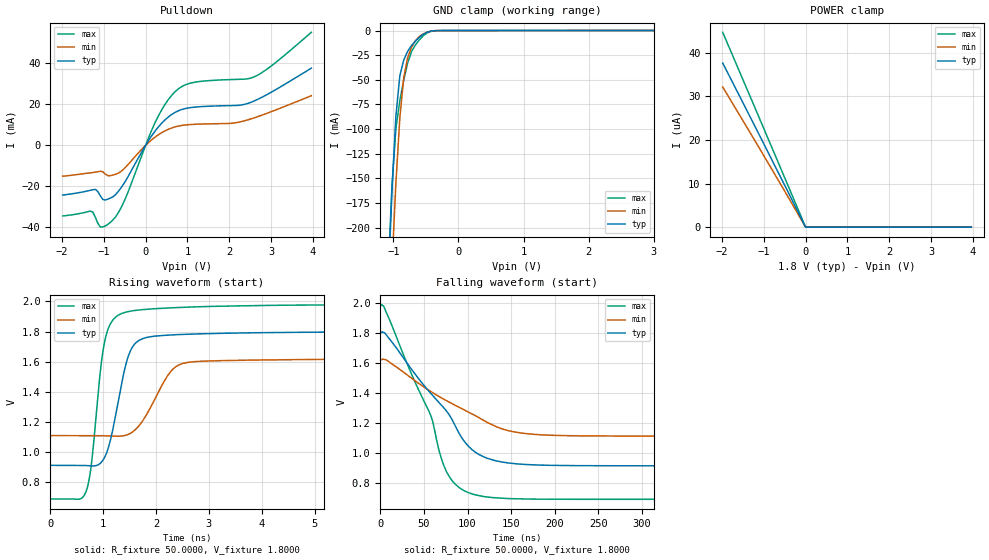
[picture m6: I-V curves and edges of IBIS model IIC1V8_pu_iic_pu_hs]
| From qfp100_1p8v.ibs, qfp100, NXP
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[Model] IIC1V8_pu_iic_pu_hs
|   Model IIC1V8_pu_iic_pu_hs
| This model was characterised for following simulation conditions:
| External (pad) voltage:
|   - Typ: 1.8V,   - Min: 1.62V,   - Max: 1.98V
| Library cells for typ/min/max conditions are connected as defined below:
|  IO - External Pad
|  A - Core Input
|  EN - Output Buffer Enable
|  BOOST - vdde
|  ECS - vdd
|  EGP - gnd
|  ENZI - vdd
|  EPD - gnd
|  EPUN - gnd
|  SSEL - vdd
|  ZI - NC
|  ZIF - NC
|  gnd - gnd
|  gnde - gnde
|  vdd - vdd
|  vdde - vdde
| All other pins connected to ground
Model_type I/O_open_drain
Polarity   Non-Inverting
Enable   Active-Low
Vinl =   0.5400V
Vinh =   1.2600V
Vmeas =  0.9000V
Cref =   0.0F
Rref =   1000.000
Vref =   1.8000V
C_comp   3.6100pF   3.4623pF   3.7513pF
|C_comp_pullup   0.9280pF   0.9063pF   0.9342pF
|C_comp_pulldown   2.3312pF   2.4847pF   2.1853pF
[Model Spec]
| variable   typ   min   max
Vinh   0.5400V   0.4860V   0.5940V
Vinl   1.2600V   1.1340V   1.3860V
Vmeas   0.9000V   0.8100V   0.9900V
Vref   1.8000V   1.6200V   1.9800V
Cref   0.0F   0.0F   0.0F
Rref   1.0000k   1.0000k   1.0000k
[Temperature Range]   25.0000   0.1250k   -40.0000
[Voltage Range]   1.8000V   1.6200V   1.9800V
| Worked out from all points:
|   slope of the pulldown table from 0 to 0.27 V, typ, clamps not added: 33.4 ohm
|   GND clamp passes 1 mA (typ) near -0.44 V on its own axis
|   rising waveform, R_fixture 50.0000, V_fixture 1.8000: 20-80 % time 318ps typ, 486ps min, 235ps max; typ from 0.912 V to 1.8 V
|   falling waveform, R_fixture 50.0000, V_fixture 1.8000: 20-80 % time 67ns typ, 88.7ns min, 48.9ns max; typ from 1.8 V to 0.912 V
[Pulldown]
|Voltage   I(typ)   I(min)   I(max)
-1.98V    -24.22mA   -15.04mA   -34.42mA
-1.32V    -21.94mA   -13.4mA    -32.06mA
-1.2V     -21.45mA   -13.05mA   -35.06mA
-1.08V    -24.63mA   -12.6mA    -39.9mA
-900mV    -26.23mA   -14.78mA   -38.53mA
-720mV    -24.07mA   -14.13mA   -34.99mA
-540mV    -19.33mA   -11.9mA    -28.53mA
300mV     8.856mA    5.096mA    14.12mA
720mV     16.26mA    9.117mA    26.48mA
1.14V     18.6mA     10.26mA    30.69mA
2.58V     21.55mA    13.34mA    33.32mA
3.96V     37.7mA     24.26mA    55.17mA
[GND_clamp]
|Voltage   I(typ)   I(min)   I(max)
-1.98V    -2.104A    -2.075A    -2.136A
-1.08V    -259.3mA   -333mA     -247mA
-1.02V    -161.8mA   -238.7mA   -157.2mA
-960mV    -86.78mA   -154.8mA   -99.51mA
-900mV    -45.99mA   -88.85mA   -71.1mA
-840mV    -29.94mA   -48.03mA   -50.31mA
-780mV    -21.2mA    -27.67mA   -33.04mA
-720mV    -15.2mA    -16.91mA   -21.32mA
-660mV    -10.61mA   -10.27mA   -14.61mA
-540mV    -3.83mA    -3.432mA   -5.346mA
-300mV    -56.31uA   -67.68uA   -68.13uA
3.96V     0A         0A         0A
[POWER_clamp]
|Voltage   I(typ)   I(min)   I(max)
-1.98V    37.59uA    32.11uA    44.63uA
-960mV    18.36uA    15.76uA    21.73uA
0V        104.7pA    4.893nA    11.38pA
3.96V     0A         0A         0A
[Ramp]
| variable   typ   min   max
dV/dt_r  0.5330/0.3182n   0.3064/0.4861n   0.7749/0.2348n
dV/dt_f  0.5329/66.9839n   0.3063/88.7255n   0.7748/48.9516n
R_load = 50.0000
[Rising Waveform]
R_fixture= 50.0000
V_fixture= 1.8000
V_fixture_min= 1.6200
V_fixture_max= 1.9800
|time   V(typ)   V(min)   V(max)
0s        911.7mV    1.109V     688.6mV
674.8ps   910.4mV    1.109V     735.9mV
774.1ps   908mV      1.11V      909mV
1.008ns   952.4mV    1.108V     1.696V
1.271ns   1.309V     1.105V     1.906V
1.478ns   1.64V      1.118V     1.933V
1.767ns   1.756V     1.218V     1.947V
2.535ns   1.782V     1.591V     1.962V
5.946ns   1.798V     1.617V     1.978V
1us       1.8V       1.62V      1.98V
[Falling Waveform]
R_fixture= 50.0000
V_fixture= 1.8000
V_fixture_min= 1.6200
V_fixture_max= 1.9800
|time   V(typ)   V(min)   V(max)
0s        1.8V       1.62V      1.98V
4.123ns   1.8V       1.623V     1.974V
58.19ns   1.393V     1.406V     1.242V
67.77ns   1.331V     1.373V     1.005V
75.75ns   1.278V     1.347V     875mV
88.71ns   1.146V     1.307V     774.7mV
112.8ns   988.9mV    1.234V     713.1mV
147.4ns   930.6mV    1.146V     693.5mV
206.1ns   914.3mV    1.114V     689.1mV
1us       911.8mV    1.109V     688.6mV
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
